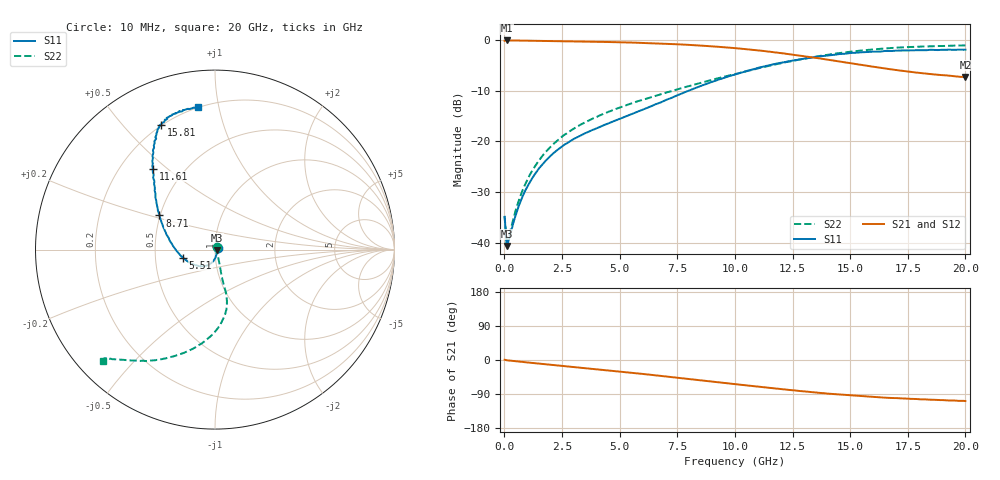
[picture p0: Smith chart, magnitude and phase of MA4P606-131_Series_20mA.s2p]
! AWR Design Environment (9226) Thu Aug 19 15:24:37 2021
! Document = '20mA'
! nPorts: 2, nXvals: 201
# GHz S DB R 50
!Freq DBS11 AngS11 DBS21 AngS21 DBS12 AngS12 DBS22 AngS22
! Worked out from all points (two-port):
!   201 points, 10 MHz to 20 GHz, reference 50 ohm
!   highest |S21| = -0.13 dB at 110 MHz (marker M1); lowest = -7.3 dB at 20 GHz (marker M2)
!   |S21| within 3 dB of the highest: start of sweep to 12.84 GHz
!   lowest |S11| = -40.6 dB at 110 MHz (marker M3), VSWR 1.02, Z = 50.9 - j0.316 ohm
!   |S11| at or under -10 dB: start of sweep to 8.017 GHz
!   |S22| runs from -40.7 to -1.1 dB; largest |S21 - S12| = 0.027
!   S11 on the Smith chart (normalised r, x): 10 MHz: 1.03, +0.01; 5.51 GHz: 0.69, -0.06; 8.71 GHz: 0.50, +0.22; 11.61 GHz: 0.34, +0.45; 15.81 GHz: 0.19, +0.64; 20 GHz: 0.20, +0.87
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0.01  -34.92 22.8  -0.19 0.7  -0.16 0.7  -34.70 45.7
0.11  -40.64 -19.6  -0.13 -0.8  -0.12 -0.7  -40.68 -20.8
0.41  -35.74 -55.1  -0.14 -2.7  -0.13 -2.7  -34.95 -51.9
0.61  -32.92 -67.2  -0.15 -4.0  -0.14 -3.9  -31.88 -59.8
0.91  -29.70 -78.3  -0.17 -5.9  -0.16 -5.7  -28.41 -65.7
1.31  -26.58 -88.4  -0.19 -8.3  -0.18 -8.1  -25.06 -69.5
1.71  -24.27 -96.4  -0.22 -10.7  -0.21 -10.5  -22.54 -71.7
2.11  -22.43 -104.0  -0.25 -13.1  -0.24 -12.8  -20.62 -73.3
2.61  -20.66 -113.2  -0.29 -16.1  -0.27 -15.7  -18.71 -74.7
3.41  -18.63 -127.5  -0.35 -20.9  -0.33 -20.3  -16.48 -75.7
4.41  -16.65 -145.9  -0.43 -26.9  -0.42 -26.3  -14.42 -76.1
5.51  -14.68 -166.0  -0.55 -33.6  -0.54 -32.8  -12.54 -75.6
6.71  -12.46 173.8  -0.72 -41.4  -0.70 -40.4  -10.85 -76.8
8.71  -8.79 148.4  -1.20 -54.7  -1.17 -53.4  -8.27 -83.1
10.01  -6.84 136.8  -1.64 -63.7  -1.59 -62.0  -6.77 -90.1
11.61  -4.90 127.5  -2.41 -74.4  -2.30 -72.7  -5.00 -102.1
13.41  -3.45 120.5  -3.50 -85.1  -3.35 -83.9  -3.39 -115.7
14.51  -2.83 116.8  -4.27 -91.0  -4.12 -90.0  -2.64 -123.0
15.81  -2.39 113.4  -5.17 -96.7  -5.07 -95.9  -1.98 -129.5
16.71  -2.23 110.5  -5.78 -100.0  -5.75 -99.1  -1.65 -132.4
19.01  -1.96 102.9  -6.96 -105.8  -7.12 -105.4  -1.23 -135.5
20  -1.94 96.9  -7.32 -108.3  -7.55 -107.1  -1.10 -135.3
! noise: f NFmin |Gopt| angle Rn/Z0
0.01  0  1  0  2e-20
2.21  0  1  0  2e-20
4.41  0  1  0  2e-20
6.61  0  1  0  2e-20
8.81  0  1  0  2e-20
11.11  0  1  0  2e-20
13.31  0  1  0  2e-20
15.51  0  1  0  2e-20
17.71  0  1  0  2e-20
20  0  1  0  2e-20
